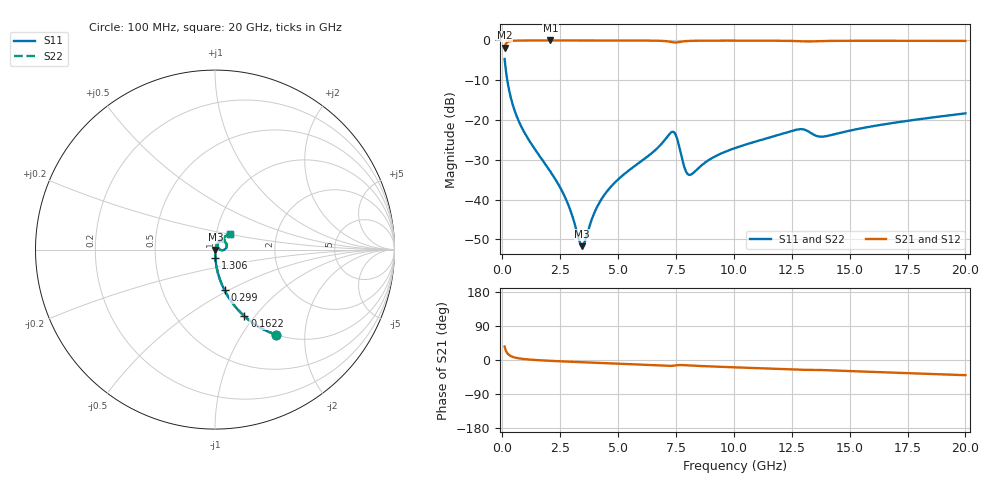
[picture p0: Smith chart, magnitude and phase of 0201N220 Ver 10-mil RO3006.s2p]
# GHz S MA R 50
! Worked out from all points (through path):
!   1601 points, 100 MHz to 20 GHz, reference 50 ohm
!   highest |S21| = -0.02 dB at 2.078 GHz (marker M1); lowest = -1.8 dB at 100 MHz (marker M2)
!   group delay of S21, straight-line fit = 6.09 ps
!   lowest |S11| = -51.7 dB at 3.446 GHz (marker M3), VSWR 1.01, Z = 50.3 - j0.0391 ohm
!   |S11| at or under -10 dB: 215.5 MHz to end of sweep
!   |S22| runs from -51.7 to -4.7 dB; largest |S21 - S12| = 0
!   S11 on the Smith chart (normalised r, x): 100 MHz: 1.00, -1.44; 162.2 MHz: 1.00, -0.89; 299 MHz: 1.00, -0.48; 1.306 GHz: 1.00, -0.10; 20 GHz: 1.16, +0.21
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0.1  0.5845 -54.3  0.8105 35.6  0.8105 35.6  0.5845 -54.3
0.1621875  0.4054 -66.2  0.9132 23.6  0.9132 23.6  0.4054 -66.2
0.299  0.2328 -76.8  0.9715 13.0  0.9715 13.0  0.2328 -76.8
0.672125  0.1028 -84.6  0.9935 4.8  0.9935 4.8  0.1028 -84.6
1.306437  0.04749 -87.6  0.9973 0.5  0.9973 0.5  0.04749 -87.6
2.077562  0.02253 -87.2  0.9977 -2.2  0.9977 -2.2  0.02253 -87.2
2.7865  0.009559 -80.2  0.9976 -4.2  0.9976 -4.2  0.009559 -80.2
3.420812  0.002629 -15.4  0.9973 -5.8  0.9973 -5.8  0.002629 -15.4
3.445688  0.002605 -8.6  0.9973 -5.8  0.9973 -5.8  0.002605 -8.6
4.03025  0.007413 60.1  0.997 -7.2  0.997 -7.2  0.007413 60.1
4.515313  0.01263 67.5  0.9967 -8.3  0.9967 -8.3  0.01263 67.5
6.741625  0.04565 63.8  0.9891 -13.9  0.9891 -13.9  0.04565 63.8
7.41325  0.07032 22.3  0.9429 -14.9  0.9429 -14.9  0.07032 22.3
7.5625  0.05673 2.8  0.9453 -13.7  0.9453 -13.7  0.05673 2.8
7.898313  0.02389 6.0  0.9773 -13.8  0.9773 -13.8  0.02389 6.0
8.097312  0.02045 29.1  0.9849 -14.4  0.9849 -14.4  0.02045 29.1
10.05  0.04443 63.0  0.9929 -19.4  0.9929 -19.4  0.04443 63.0
12.71162  0.07569 51.2  0.9796 -25.5  0.9796 -25.5  0.07569 51.2
13.37081  0.0675 40.4  0.9706 -25.9  0.9706 -25.9  0.0675 40.4
13.90563  0.06213 48.3  0.9817 -26.7  0.9817 -26.7  0.06213 48.3
16.69162  0.09018 52.6  0.9886 -32.9  0.9886 -32.9  0.09018 52.6
20  0.1212 46.7  0.9853 -40.1  0.9853 -40.1  0.1212 46.7
